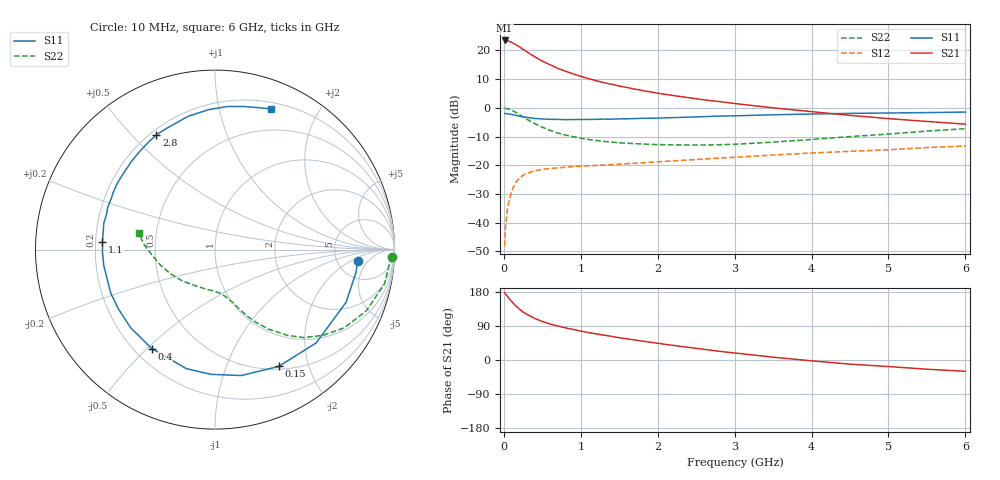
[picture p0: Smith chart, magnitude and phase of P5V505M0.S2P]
! SIEMENS Small Signal Semiconductors
! BFP183
! Si NPN RF Bipolar Junction Transistor in SOT143
! VCE = 0.5 V  IC = 5 mA
! Common Emitter S-Parameters:  March  1996
# GHz  S  MA  R  50
!  f  S11  S21  S12  S22
! GHz  MAG  ANG  MAG  ANG  MAG  ANG  MAG  ANG
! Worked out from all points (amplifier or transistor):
!   36 points, 10 MHz to 6 GHz, reference 50 ohm
!   highest |S21| = 23.5 dB at 10 MHz (marker M1)
!   |S21| within 3 dB of that: start of sweep to 244.7 MHz
!   unconditionally stable (mu >= 1): 1.352 GHz to end of sweep
!   at 250 MHz: K = 0.23, MSG = 21.9 dB, |S12| = -23.5 dB
!   at 1.4 GHz: K = 1.03, MAG = 13.0 dB, |S12| = -19.8 dB
!   at 6 GHz: K = 1.15, MAG = 1.4 dB, |S12| = -13.3 dB
!   S11 on the Smith chart (normalised r, x): 10 MHz: 7.91, -2.71; 150 MHz: 0.54, -1.55; 400 MHz: 0.27, -0.52; 1.1 GHz: 0.23, +0.03; 2.8 GHz: 0.22, +0.59; 6 GHz: 0.26, +1.44
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0.01  0.7971 -4.5  14.92 177.6  0.0039 86.9  0.985 -2.3
0.02  0.7961 -9.0  14.9 175.2  0.0079 85.4  0.9748 -4.7
0.05  0.7871 -21.9  14.66 166.9  0.019 79.6  0.9639 -11.4
0.1  0.7669 -42.6  13.83 154.8  0.0354 68.4  0.9094 -22.0
0.15  0.7416 -61.3  12.73 143.9  0.0494 59.4  0.8418 -31.2
0.2  0.7169 -78.2  11.61 134.6  0.0595 52.2  0.7678 -38.5
0.25  0.6953 -91.9  10.44 126.7  0.0669 46.2  0.6953 -44.8
0.3  0.6821 -103.5  9.461 120.6  0.0725 42.0  0.6311 -49.4
0.4  0.6545 -122.6  7.774 109.7  0.0804 35.3  0.533 -56.2
0.5  0.6405 -137.1  6.507 101.7  0.085 30.9  0.4594 -61.0
0.6  0.6318 -148.3  5.637 95.2  0.088 28.2  0.4046 -64.6
0.7  0.6294 -157.4  4.878 89.8  0.0898 26.6  0.365 -67.2
0.9  0.626 -171.7  3.908 80.7  0.0947 24.5  0.3148 -71.1
1.1  0.6284 176.1  3.236 72.4  0.0979 23.3  0.2813 -75.2
1.5  0.6425 158.5  2.401 58.8  0.1043 23.1  0.246 -82.7
1.8  0.6566 146.9  2.008 49.9  0.1105 23.2  0.2347 -88.8
2.2  0.676 133.8  1.64 38.6  0.1191 22.8  0.2269 -99.0
2.8  0.7182 117.0  1.283 23.0  0.1332 22.1  0.2282 -116.1
3.5  0.7573 101.5  1 7.5  0.1509 19.8  0.2529 -136.7
4.5  0.8009 84.7  0.74 -10.9  0.175 14.6  0.3158 -163.9
5.5  0.8263 73.2  0.58 -24.3  0.2035 9.6  0.3936 176.5
6  0.8444 68.2  0.52 -29.8  0.2162 5.5  0.4341 167.9
